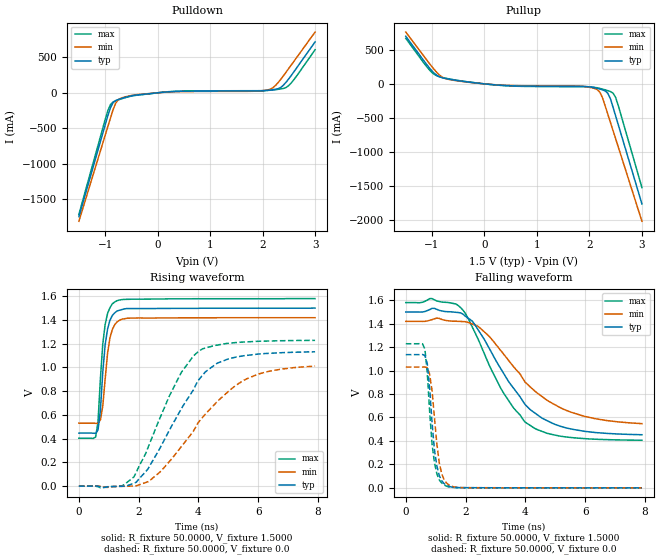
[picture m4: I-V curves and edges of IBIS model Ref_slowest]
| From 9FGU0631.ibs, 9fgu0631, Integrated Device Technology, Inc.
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[Model]  Ref_slowest
Model_type Output
Polarity   Non-Inverting
Enable   Active-High
Vmeas =  0.9000V
Cref =   5.0000pF
Rref =   0.0
Vref =   0.9000V
C_comp   1.1000pF   1.0000pF   1.2000pF
[Temperature Range]   25.0000   75.0000   0.0
[Voltage Range]   1.5000V   1.4200V   1.5800V
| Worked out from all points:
|   slope of the pulldown table from 0 to 0.225 V, typ, clamps not added: 15.7 ohm
|   slope of the pullup table from 0 to 0.225 V, typ, clamps not added: 14.4 ohm
|   rising waveform, R_fixture 50.0000, V_fixture 1.5000: 20-80 % time 214ps typ, 223ps min, 209ps max; typ from 0.446 V to 1.5 V
|   rising waveform, R_fixture 50.0000, V_fixture 0.0: 20-80 % time 1.54ns typ, 2.04ns min, 1.32ns max; typ from 0 V to 1.13 V
|   falling waveform, R_fixture 50.0000, V_fixture 1.5000: 20-80 % time 1.62ns typ, 1.95ns min, 1.48ns max; typ from 1.5 V to 0.453 V
|   falling waveform, R_fixture 50.0000, V_fixture 0.0: 20-80 % time 240ps typ, 247ps min, 226ps max; typ from 1.14 V to 0 V
[Pulldown]
|Voltage   I(typ)   I(min)   I(max)
-1.5V     -1.745A    -1.809A    -1.713A
-950mV    -327.8mA   -480.1mA   -255.7mA
-900mV    -212.5mA   -359.3mA   -168.3mA
-850mV    -140.3mA   -241.1mA   -129.4mA
-750mV    -94.02mA   -98.51mA   -100.2mA
-450mV    -36.28mA   -31.57mA   -39.68mA
250mV     15.41mA    12.24mA    17.86mA
1.8V      25.49mA    21.55mA    29.47mA
2.15V     39.17mA    51.36mA    36.57mA
2.35V     77.57mA    193.2mA    55.3mA
2.5V      197.9mA    344.2mA    103.1mA
3V        716.8mA    855.6mA    606.3mA
[Pullup]
|Voltage   I(typ)   I(min)   I(max)
-1.5V     699.4mA    760.9mA    669.2mA
-1V       189.6mA    251.3mA    166.1mA
-900mV    121.4mA    161.2mA    115.6mA
-750mV    80mA       79.09mA    84.43mA
350mV     -22.11mA   -19.15mA   -24.57mA
1.8V      -36.31mA   -32.03mA   -41.75mA
2.15V     -66.71mA   -84.88mA   -58.33mA
2.25V     -87.88mA   -207.1mA   -76.93mA
2.35V     -137.7mA   -445.8mA   -99.43mA
2.45V     -344.5mA   -687.2mA   -135.9mA
2.5V      -473.4mA   -808mA     -201.5mA
3V        -1.763A    -2.017A    -1.522A
[Ramp]
| variable   typ   min   max
dV/dt_r  0.6792/1.6026n   0.6066/2.0935n   0.7368/1.3047n
dV/dt_f  0.6283/1.6821n   0.5234/2.0049n   0.7045/1.4576n
R_load = 50.0000
[Rising Waveform]
R_fixture= 50.0000
V_fixture= 1.5000
V_fixture_min= 1.4200
V_fixture_max= 1.5800
|time   V(typ)   V(min)   V(max)
0s        446.5mV    530.1mV    403.2mV
560ps     444.3mV    528.6mV    412.9mV
640ps     472.4mV    528.2mV    540.4mV
720ps     637.8mV    557.7mV    905.2mV
800ps     963.3mV    676.6mV    1.2V
880ps     1.194V     904.4mV    1.364V
1.04ns    1.398V     1.251V     1.504V
1.2ns     1.46V      1.36V      1.552V
1.76ns    1.496V     1.416V     1.575V
7.9ns     1.5V       1.419V     1.58V
[Rising Waveform]
R_fixture= 50.0000
V_fixture= 0.0
V_fixture_min= 0.0
V_fixture_max= 0.0
|time   V(typ)   V(min)   V(max)
0s        0V         0V         0V
1.44ns    -1.83mV    -2.286mV   1.075mV
1.84ns    23.2mV     952.9uV    77.02mV
2.31ns    144.2mV    36.49mV    322.9mV
2.71ns    318.6mV    117.1mV    572.4mV
3.43ns    652.2mV    333.3mV    959.5mV
4.07ns    914.2mV    558.8mV    1.146V
4.63ns    1.036V     712.7mV    1.188V
5.59ns    1.101V     901.4mV    1.215V
7.9ns     1.132V     1.011V     1.228V
[Falling Waveform]
R_fixture= 50.0000
V_fixture= 1.5000
V_fixture_min= 1.4200
V_fixture_max= 1.5800
|time   V(typ)   V(min)   V(max)
0s        1.5V       1.42V      1.58V
880ps     1.531V     1.435V     1.614V
1.84ns    1.492V     1.419V     1.536V
2.47ns    1.328V     1.367V     1.239V
3.27ns    977.7mV    1.142V     809.7mV
3.99ns    711mV      902.5mV    561.1mV
4.31ns    639.6mV    826.5mV    507.4mV
4.95ns    545.5mV    714.3mV    452.4mV
5.91ns    484.9mV    615mV      421.1mV
7.9ns     452.9mV    547.6mV    405.9mV
[Falling Waveform]
R_fixture= 50.0000
V_fixture= 0.0
V_fixture_min= 0.0
V_fixture_max= 0.0
|time   V(typ)   V(min)   V(max)
0s        1.136V     1.03V      1.229V
640ps     1.129V     1.031V     1.184V
720ps     1.059V     1.024V     979.1mV
800ps     845.7mV    969.1mV    645.6mV
880ps     555.4mV    827.1mV    372.9mV
960ps     321.9mV    597.8mV    214.4mV
1.12ns    105.9mV    215.2mV    68.17mV
1.28ns    36.69mV    71.26mV    24.1mV
1.76ns    2.096mV    2.809mV    1.487mV
7.9ns     7.042uV    17.01uV    3.539uV
